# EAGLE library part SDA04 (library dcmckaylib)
DIP Switch (SPST) x 4
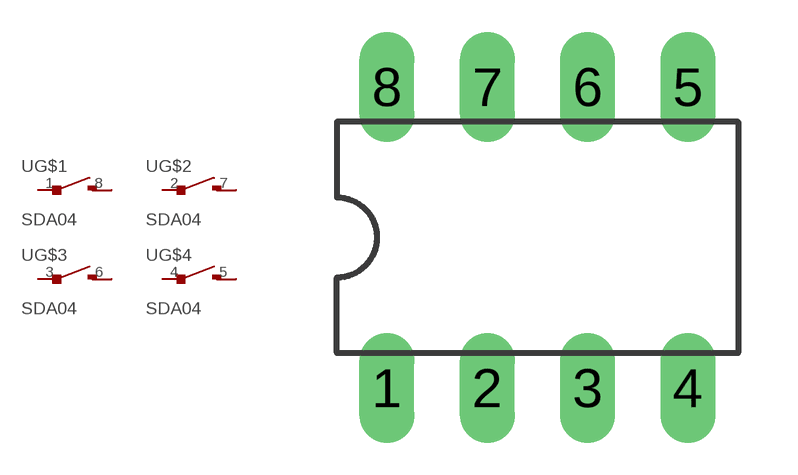
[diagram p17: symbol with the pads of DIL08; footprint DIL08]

Designator prefix -; gates G$1=SPSTSWITCH2 G$2=SPSTSWITCH2 G$3=SPSTSWITCH2 G$4=SPSTSWITCH2

## SDA04  [DIL08]
1  G$1:P$1
2  G$2:P$1
3  G$3:P$1
4  G$4:P$1
5  G$4:P$3
6  G$3:P$3
7  G$2:P$3
8  G$1:P$3

## Footprint DIL08 (pad centres in mm)
Dual In Line Package
drill 0.889 long: 1 -3.81,-3.81; 2 -1.27,-3.81; 3 1.27,-3.81; 4 3.81,-3.81; 5 3.81,3.81; 6 1.27,3.81; 7 -1.27,3.81; 8 -3.81,3.81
